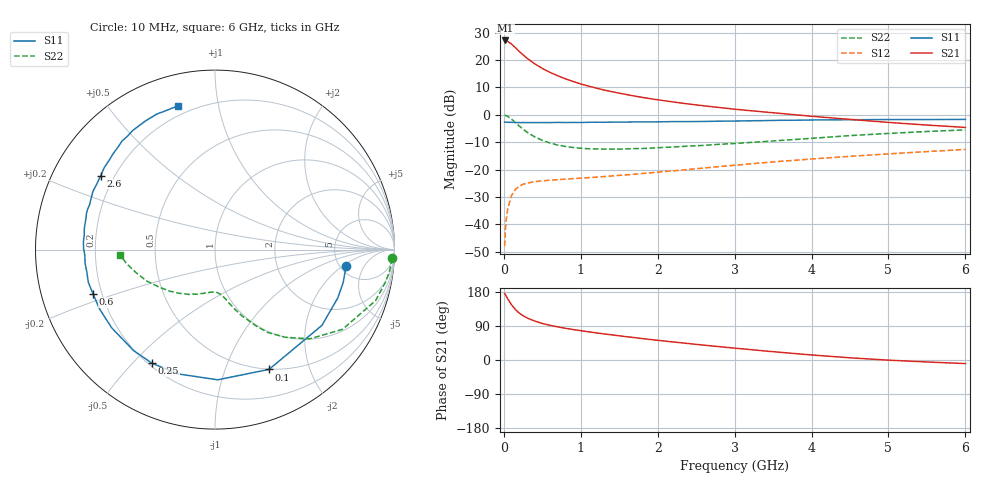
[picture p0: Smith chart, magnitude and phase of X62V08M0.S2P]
! SIEMENS Small Signal Semiconductors
! BFP193W
! Si NPN RF Bipolar Junction Transistor in SOT343
! VCE = 2 V  IC = 8 mA
! Common Emitter S-Parameters:  April 1994
# GHz  S  MA  R  50
!  f  S11  S21  S12  S22
! GHz  MAG  ANG  MAG  ANG  MAG  ANG  MAG  ANG
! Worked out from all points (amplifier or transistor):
!   40 points, 10 MHz to 6 GHz, reference 50 ohm
!   highest |S21| = 27.2 dB at 20 MHz (marker M1)
!   |S21| within 3 dB of that: start of sweep to 163.9 MHz
!   unconditionally stable (mu >= 1): 1.405 GHz to 4.352 GHz
!   at 200 MHz: K = 0.19, MSG = 24.6 dB, |S12| = -26.1 dB
!   at 1.5 GHz: K = 1.04, MAG = 13.9 dB, |S12| = -22.1 dB
!   at 6 GHz: K = 0.94, MSG = 4.0 dB, |S12| = -12.6 dB
!   lowest NFmin = 1.25 dB at 450 MHz
!   S11 on the Smith chart (normalised r, x): 10 MHz: 5.68, -2.23; 100 MHz: 0.50, -1.43; 250 MHz: 0.21, -0.57; 600 MHz: 0.17, -0.17; 2.6 GHz: 0.15, +0.29; 6 GHz: 0.15, +0.76
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0.01  0.7361 -7.0  22.82 175.4  0.004 87.0  0.9869 -2.8
0.02  0.7375 -14.4  22.86 172.5  0.0078 82.7  0.9794 -7.3
0.03  0.7351 -21.5  22.64 168.8  0.0118 81.1  0.967 -10.8
0.05  0.7303 -35.3  22 161.5  0.0192 73.1  0.9388 -17.6
0.1  0.7323 -65.7  19.6 145.8  0.0338 59.7  0.8381 -32.0
0.15  0.7256 -88.8  16.92 133.1  0.0435 49.7  0.7251 -43.3
0.2  0.7223 -106.4  14.43 123.9  0.0497 42.8  0.6258 -51.3
0.25  0.724 -119.0  12.51 116.8  0.0542 38.1  0.5486 -57.4
0.3  0.7227 -129.0  10.85 111.2  0.0567 34.5  0.4832 -61.7
0.4  0.722 -142.9  8.59 102.8  0.0602 30.5  0.3975 -67.9
0.5  0.7232 -152.8  7.056 96.4  0.0625 28.6  0.3431 -72.2
0.6  0.7228 -160.0  5.963 91.5  0.064 27.6  0.3061 -75.5
0.8  0.7248 -170.2  4.554 83.7  0.067 28.4  0.2651 -80.3
1.1  0.7321 179.5  3.36 74.4  0.0714 30.4  0.2401 -86.5
1.3  0.7328 173.8  2.851 68.9  0.0747 32.7  0.2373 -90.5
1.6  0.7393 166.5  2.343 61.3  0.0803 35.9  0.239 -96.2
2.2  0.7535 154.5  1.723 47.6  0.095 40.6  0.2585 -108.5
2.6  0.7585 147.1  1.463 39.2  0.1069 42.7  0.2773 -116.9
3.2  0.7789 136.9  1.194 27.6  0.1273 43.7  0.3134 -129.0
4.5  0.815 118.4  0.827 5.8  0.1749 40.7  0.4179 -155.1
5.5  0.8212 109.2  0.652 -5.2  0.2135 36.0  0.4972 -170.7
6  0.8269 104.6  0.59 -9.4  0.2338 33.6  0.5321 -177.0
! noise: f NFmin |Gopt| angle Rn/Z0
0.45  1.25  0.23  133  0.12
0.9  1.3  0.35  156  0.11
1.8  2  0.55  -155  0.13
